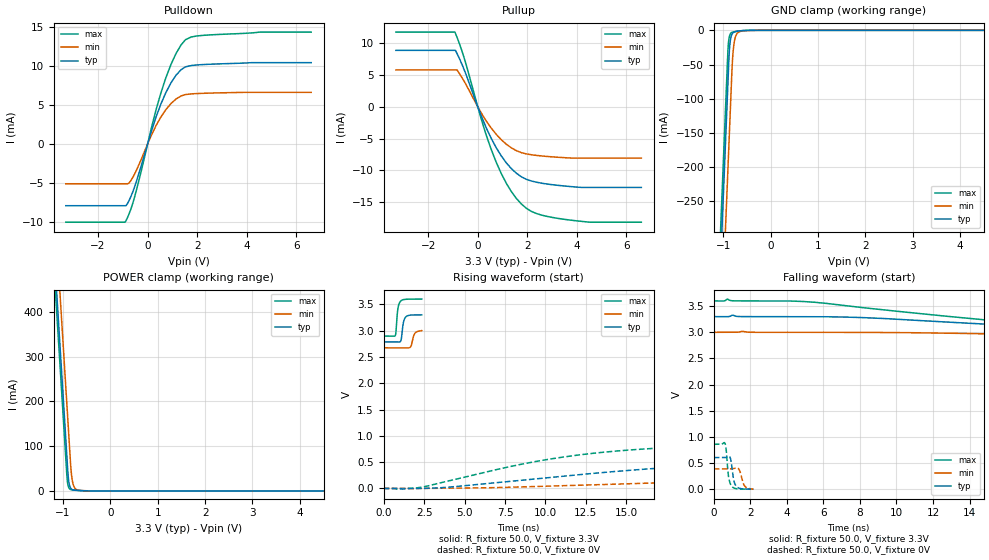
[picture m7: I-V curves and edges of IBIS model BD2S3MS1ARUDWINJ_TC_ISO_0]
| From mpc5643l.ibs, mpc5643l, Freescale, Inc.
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| *** New cell (Generated with 5.14beta1 (Sep 20 2010 13:23:23))
[Model]   BD2S3MS1ARUDWINJ_TC_ISO_0
Model_type I/O
Polarity   Non-Inverting
Enable   Active-Low
| CAP_THRESHOLD on pad pad is "CMOS" :
| Rising=10.0% of VDDE1   Falling=90.0% of VDDE1
| C_comp min and max val. don't necessarily correlate with the min and max pvt
| but are the smallest and greatest pad capacitance found.
| var   typ   min   max
C_comp   1.61143pF  1.53237pF  1.70132pF
Vinl = 1.05V | Dummy value overriden by next lines
Vinh = 2.34V | Dummy value overriden by next lines
Vmeas = 1.65V   | Reference voltage for timing measurements
Cref  = 25.0pF   | Timing specification test load capacitance value
Rref  = 1.0MOhm   | Timing specification test load resistance value
Vref  = 1.65V   | Timing specification test load voltage
[Model Spec]
| TIME_THRESHOLD on pin ipp_ind is "CORE" :
| Rising=40.0% of VDD   Falling=60.0% of VDD
Vinl 1.30950V 1.19650V 1.40650V
Vinh 1.89650V 1.72150V 2.04550V
| variable   typ   min   max
[Temperature Range] 25.0 150.0 -40.0
| variable   typ   min   max
[Voltage Range] 3.3V 3.0V 3.6V
| variable   typ   min   max
[POWER Clamp Reference] 3.3V 3.0V 3.6V
| variable   typ   min   max
[GND Clamp Reference] 0V 0V 0V
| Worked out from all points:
|   slope of the pulldown table from 0 to 0.495 V, typ, clamps not added: 104 ohm
|   slope of the pullup table from 0 to 0.495 V, typ, clamps not added: 108 ohm
|   GND clamp passes 1 mA (typ) near -0.66 V on its own axis
|   POWER clamp passes 1 mA (typ) near -0.67 V on its own axis
|   rising waveform, R_fixture 50.0, V_fixture 3.3V: 20-80 % time 144ps typ, 173ps min, 128ps max; typ from 2.79 V to 3.3 V
|   falling waveform, R_fixture 50.0, V_fixture 3.3V: 20-80 % time 19.3ns typ, 30.3ns min, 13.8ns max; typ from 3.3 V to 2.79 V
|   rising waveform, R_fixture 50.0, V_fixture 0V: 20-80 % time 15.5ns typ, 30.8ns min, 9.12ns max; typ from 0 V to 0.604 V
|   falling waveform, R_fixture 50.0, V_fixture 0V: 20-80 % time 166ps typ, 200ps min, 149ps max; typ from 0.604 V to 0 V
[POWER Clamp]
-3.3V     4.126A     4.242A     4.083A
-1.21V    573.2mA    689.5mA    530.1mA
-1.14V    454.2mA    570.5mA    411.1mA
-1.07V    335.2mA    451.5mA    292.1mA
-1V       216.2mA    332.5mA    173.1mA
-910mV    63.16mA    179.5mA    23.78mA
-880mV    22.46mA    128.5mA    7.535mA
-840mV    6.363mA    60.49mA    3.143mA
-810mV    3.226mA    27.5mA     2.363mA
-770mV    1.895mA    10.15mA    1.875mA
-620mV    704.1uA    944.2uA    740.5uA
6.6V      0A         0A         0A
[GND Clamp]
-3.3V     -4.155A    -4.281A    -4.106A
-1.08V    -381.1mA   -506.9mA   -332.4mA
-910mV    -92.11mA   -217.9mA   -43.37mA
-890mV    -58.11mA   -183.9mA   -18.27mA
-870mV    -28.8mA    -149.9mA   -8.794mA
-850mV    -14.7mA    -115.9mA   -5.11mA
-810mV    -4.921mA   -49.94mA   -2.835mA
-780mV    -2.872mA   -23.15mA   -2.229mA
-740mV    -1.846mA   -8.915mA   -1.687mA
-680mV    -1.151mA   -2.788mA   -1.045mA
-560mV    -368.5uA   -711.5uA   -256.2uA
6.6V      11.35nA    2.808uA    94.32pA
| variable   typ   min   max
[Pullup Reference] 3.3V 3.0V 3.6V
| variable   typ   min   max
[Pulldown Reference] 0V 0V 0V
[Pullup]
-3.3V     8.847mA    5.784mA    11.72mA
-920mV    8.847mA    5.784mA    11.72mA
-840mV    8.382mA    5.784mA    10.94mA
-530mV    5.641mA    3.871mA    7.427mA
340mV     -3.289mA   -2.224mA   -4.425mA
740mV     -6.399mA   -4.306mA   -8.659mA
950mV     -7.722mA   -5.179mA   -10.49mA
1.35V     -9.688mA   -6.439mA   -13.28mA
1.96V     -11.39mA   -7.41mA    -15.93mA
2.57V     -12mA      -7.725mA   -17mA
3.78V     -12.54mA   -8.06mA    -17.82mA
6.6V      -12.67mA   -8.069mA   -18.12mA
[Pulldown]
-3.3V     -7.921mA   -5.109mA   -10.04mA
-900mV    -7.921mA   -5.109mA   -9.995mA
-750mV    -7.258mA   -4.993mA   -8.98mA
-540mV    -5.638mA   -3.948mA   -6.973mA
340mV     3.462mA    2.363mA    4.387mA
740mV     6.62mA     4.428mA    8.533mA
1.15V     8.842mA    5.781mA    11.64mA
1.35V     9.537mA    6.164mA    12.71mA
1.55V     9.918mA    6.352mA    13.42mA
1.96V     10.14mA    6.469mA    13.85mA
2.57V     10.25mA    6.538mA    14.01mA
6.6V      10.44mA    6.628mA    14.36mA
[Ramp]
dV/dt_r 362.31448mV/15.47884ns 232.21452mV/30.76292ns 515.1225mV/9.12252ns
dV/dt_f 308.17507mV/19.30155ns 196.13077mV/30.31686ns 422.03899mV/13.81311ns
R_load = 50.0
| Removed startup time: 0s 0s 0s  .
| Removed end time: 2.355ns.
[Rising Waveform]
R_fixture   = 50.0
V_fixture   = 3.3V
V_fixture_min = 3.0V
V_fixture_max = 3.6V
0s        2.786V     2.673V     2.897V
721ps     2.786V     2.673V     2.907V
761ps     2.786V     2.673V     2.973V
880ps     2.785V     2.673V     3.416V
1.063ns   2.807V     2.673V     3.566V
1.216ns   3.147V     2.673V     3.588V
1.354ns   3.256V     2.672V     3.595V
1.675ns   3.295V     2.695V     3.598V
1.957ns   3.299V     2.958V     3.599V
2.357ns   3.3V       3V         3.6V
| Removed startup time: 0s 0s 0s  .
| Removed end time: 130.7ns.
[Falling Waveform]
R_fixture   = 50.0
V_fixture   = 3.3V
V_fixture_min = 3.0V
V_fixture_max = 3.6V
0s        3.3V       3V         3.6V
750ps     3.299V     3V         3.636V
1.1ns     3.32V      2.999V     3.602V
5.2ns     3.3V       3V         3.583V
8.75ns    3.273V     2.998V     3.449V
19.5ns    3.072V     2.935V     3.102V
29.55ns   2.916V     2.859V     2.952V
40.55ns   2.837V     2.783V     2.918V
60.15ns   2.802V     2.714V     2.902V
130.8ns   2.786V     2.673V     2.897V
| Removed startup time: 0s 0s 0s  .
| Removed end time: 109.0ns.
[Rising Waveform]
R_fixture   = 50.0
V_fixture   = 0V
V_fixture_min = 0V
V_fixture_max = 0V
0s        15.94nV    1.092uV    14.27nV
800ps     172.1uV    1.164uV    -14.16mV
2.4ns     874.9uV    -220.2uV   26.14mV
8.1ns     142.3mV    25.16mV    434mV
12.1ns    262.1mV    60.18mV    637.6mV
16.15ns   366.6mV    98.08mV    750.9mV
21.1ns    459mV      146.1mV    813.6mV
32.3ns    559.1mV    240.9mV    851.5mV
50.75ns   596.7mV    331mV      857.9mV
109.1ns   603.9mV    387mV      858.5mV
| Removed startup time: 0s 0s 0s  .
| Removed end time: 2.164ns.
[Falling Waveform]
R_fixture   = 50.0
V_fixture   = 0V
V_fixture_min = 0V
V_fixture_max = 0V
0s        603.9mV    387.1mV    858.5mV
617ps     603.8mV    387.1mV    874.3mV
676ps     608.6mV    387.1mV    767.1mV
812ps     631.9mV    386.9mV    233.6mV
990ps     425.8mV    388.1mV    51.82mV
1.103ns   158.8mV    395.9mV    22.9mV
1.256ns   46.71mV    407.8mV    8.222mV
1.413ns   15.92mV    357.1mV    3.351mV
1.697ns   3.132mV    58.43mV    927.9uV
2.166ns   67.82uV    42.03uV    135uV
